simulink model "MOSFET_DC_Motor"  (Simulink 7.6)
settings: Solver=ode23tb  StartTime=0.0  StopTime=5  RelTol=1e-4
InitFcn:
  | Couple=50;
  | ton=0.5;
  | toff=3;
StopFcn:
  | close all
  | load MOSFET.mat
  | plotyy(x(1,:),x(2,:), x(1,:),x(3,:))
  | grid
  | title('Vitesse moteur et courant armature')
  | xlabel('temps')
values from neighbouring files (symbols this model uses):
  A = [1+j -(1-j);1 -2/(1-j)]    [systeme_AX_B_phaseurs.m]
  N = 50;')    [Prog_callbacks.m]    (also in _startup.m = 0.001'))
undefined symbols (not defined in the file or in its folder): constant, Torque
libraries: powerlib x6, simulink x2, powerlib_extras x1

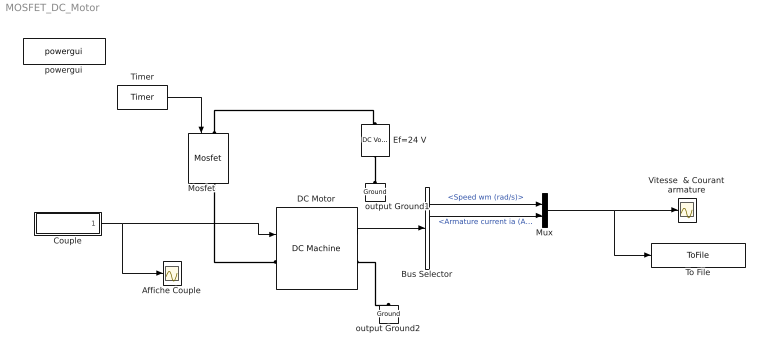
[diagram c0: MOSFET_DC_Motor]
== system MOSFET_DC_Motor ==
  Affiche Couple : Scope
  Bus Selector : BusSelector  OutputSignals=Speed wm (rad/s),Armature current ia (A),Field current if (A),Electrical torque Te (n m)
  Couple : Subsystem
  DC Motor : powerlib/Machines/DC Machine  DialogController=POWERSYS.PowerSysDialog  SystemSampleTime=-1  PresetModel=No  MechanicalLoad=Torque TL  FieldType=Permanent magnet  ShowDetailedParameters=on  RLa="[ 0.6  0.012]"  RLf="[ 240  120]"  Laf=1.8  MachineConstant=Torque constant (N.m/A)  Ke=1.8  Kt=1.8  J=1  Bm=0  Tf=0  w0=0  Ifinit=1  TsPowergui=0  TsBlock=-1
  Ef=24 V : powerlib/Electrical Sources/DC Voltage Source  Description=source block  DialogController=POWERSYS.PowerSysDialog  SystemSampleTime=-1  Amplitude=24  Measurements=None
  Mosfet : powerlib/Power Electronics/Mosfet  DialogController=POWERSYS.PowerSysDialog  SystemSampleTime=-1  Ron=0.1  Lon=0  Rd=0.01  Vfd=0  IC=0  Rs=1e5  Cs=inf  Measurements=on
  Mux : Mux  Inputs=2
  Timer : powerlib_extras/Control  Blocks/Timer  DialogController=POWERSYS.PowerSysDialog  SystemSampleTime=-1  t=[0 1]  e=[0 1]
  To File : ToFile  Filename=MOSFET  MatrixName=x
  Vitesse  & Courant armature : Scope
  output Ground1 : powerlib/Elements/Ground  DialogController=POWERSYS.PowerSysDialog  PhysicalDomain=powersysdomain  SubClassName=unknown  LeftPortType=p1  RightPortType=p1  LConnTagsString=a
  output Ground2 : powerlib/Elements/Ground  DialogController=POWERSYS.PowerSysDialog  PhysicalDomain=powersysdomain  SubClassName=unknown  LeftPortType=p1  RightPortType=p1  LConnTagsString=a
  powergui : powerlib/powergui  Priority=2  SystemSampleTime=-1  SimulationMode=Continuous  SampleTime=0  frequency=60  SPID=off  DisableSnubberDevices=off  DisableRonSwitches=off  DisableVfSwitches=off  SwTol=0  Interpol=off  frequencyindice=0  echomessages=off  HookPort=off  DisplayEquations=off  FunctionMessages=off  EnableUseOfTLC=off  x0status=blocks  RestoreLinks=warning  ResistiveCurrentMeasurement=off  Frange=logspace(0,3,50)  Ylog=off  Xlog=off  ShowGrid=off  save=off  variable=ZData  ZoomFFT=on  StartTime=0.0  cycles=1  DisplayStyle=off  fundamental=60  FreqAxis=off  MaxFrequency=1000  frequencyindicesteady=1  RmsSteady=1  display=off  Ts=0  methode=off
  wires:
  Timer/1 -> Mosfet/1
  Bus Selector/1 -> Mux/1  "<Speed wm (rad/s)>"
  Mux/1 -> Vitesse  & Courant armature/1, To File/1
  Couple/1(Out1) -> Affiche Couple/1, DC Motor/1
  DC Motor/1 -> Bus Selector/1
  Bus Selector/2 -> Mux/2  "<Armature current ia (A)>"
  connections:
  Ef=24 V/LConn1 -- output Ground1/LConn1
  Mosfet/LConn1 -- Ef=24 V/RConn1
  Mosfet/RConn1 -- DC Motor/LConn1
  DC Motor/RConn1 -- output Ground2/LConn1

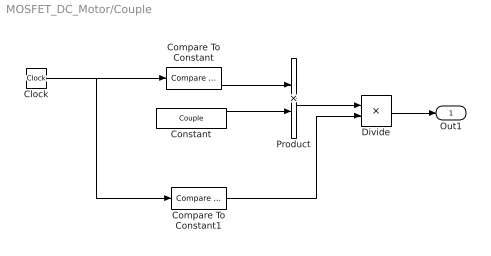
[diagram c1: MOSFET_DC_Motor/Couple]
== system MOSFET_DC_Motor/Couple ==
  Clock : Clock
  Compare To Constant : simulink/Logic and Bit Operations/Compare To Constant  SystemSampleTime=-1  relop=>=  const=ton  LogicOutDataTypeMode=uint8
  Compare To Constant1 : simulink/Logic and Bit Operations/Compare To Constant  SystemSampleTime=-1  relop=>=  const=toff  LogicOutDataTypeMode=uint8
  Constant : Constant  Value=Couple
  Divide : Product  Inputs=**
  Product : Product
  Out1 : Outport
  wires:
  Clock/1 -> Compare To Constant/1, Compare To Constant1/1
  Compare To Constant/1 -> Product/1
  Constant/1 -> Product/2
  Product/1 -> Divide/1
  Compare To Constant1/1 -> Divide/2
  Divide/1 -> Out1/1
